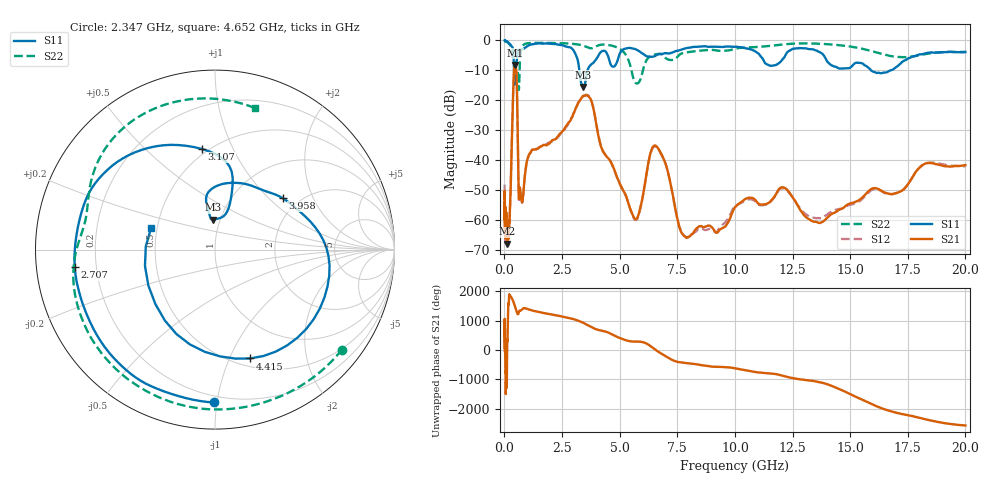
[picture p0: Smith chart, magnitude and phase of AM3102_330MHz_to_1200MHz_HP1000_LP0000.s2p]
! Date/Time: Tue, Sep 11, 2018 5:16 PM
! Network Analyzer: Agilent Technologies E8362B Rev: A.07.50.63
! Sweep from 0.010 to 20.000 GHz, 1601 Points, Sweep Type: LOG
! Power Supply: 4.949 V, 0.001 A
# Hz S DB R 50
!freq MagS11 AngS11 MagS21 AngS21 MagS12 AngS12 MagS22 AngS22
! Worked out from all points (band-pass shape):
!   1601 points, 10 MHz to 20 GHz, reference 50 ohm
!   highest |S21| = -8.17 dB at 455.8 MHz (marker M1); lowest = -67.8 dB at 118.3 MHz (marker M2)
!   |S21| within 3 dB of the highest: 410.5 MHz to 524.4 MHz (113.9 MHz wide, 24.4 % of centre)
!   lowest |S11| = -15.5 dB at 3.432 GHz (marker M3), VSWR 1.40, Z = 46.5 + j16 ohm
!   |S11| at or under -10 dB: 417 MHz to 463.4 MHz (46.46 MHz wide, 10.6 % of centre); 3.251 GHz to 3.606 GHz (354.6 MHz wide, 10.3 % of centre); 15.91 GHz to 16.76 GHz (846.5 MHz wide, 5.18 % of centre)
!   |S22| runs from -16.5 to -0.1 dB; largest |S21 - S12| = 0.006
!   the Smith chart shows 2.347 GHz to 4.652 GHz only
!   S11 on the Smith chart (normalised r, x): 2.347 GHz: 0.16, -0.98; 2.707 GHz: 0.12, -0.06; 3.107 GHz: 0.47, +0.77; 3.958 GHz: 1.65, +1.22; 4.415 GHz: 0.58, -1.19; 4.652 GHz: 0.46, +0.13
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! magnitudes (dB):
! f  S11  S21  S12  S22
! 10 MHz  0.0  -52.6  -48.1  -0.1
! 35.55 MHz  0.0  -62.5  -64.5  -0.2
! 118.3 MHz  -0.3  -67.8  -63.3  -0.6
! 126.4 MHz  -0.4  -64.9  -63.8  -0.6
! 236.6 MHz  -1.1  -57.3  -58.1  -1.4
! 447.2 MHz  -14.1  -8.2  -8.3  -6.4
! 455.8 MHz  -12.1  -8.2  -8.2  -6.5
! 533.2 MHz  -7.1  -12.9  -12.9  -12.1
! 632.6 MHz  -3.1  -52.9  -53.1  -16.2
! 757.7 MHz  -2.9  -53.8  -53.9  -2.3
! 1.59 GHz  -1.0  -35.3  -35.3  -0.8
! 2.347 GHz  -1.4  -31.7  -32.1  -0.9
! 2.707 GHz  -2.1  -28.2  -28.7  -1.0
! 3.107 GHz  -5.0  -22.3  -22.5  -1.2
! 3.432 GHz  -15.5  -18.5  -18.6  -1.8
! 3.958 GHz  -6.5  -26.7  -26.5  -2.1
! 4.415 GHz  -3.9  -38.6  -38.5  -1.4
! 4.652 GHz  -8.5  -41.0  -41.2  -1.7
! 5.652 GHz  -2.8  -59.5  -59.8  -13.7
! 6.549 GHz  -5.1  -35.1  -35.3  -4.6
! 7.92 GHz  -2.5  -65.8  -65.9  -3.9
! 20 GHz  -3.9  -41.6  -42.1  -3.8
